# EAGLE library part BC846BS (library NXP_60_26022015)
Dual 65 V, 100 mA NPN/NPN general-purpose transistor AAL Eindhoven MK
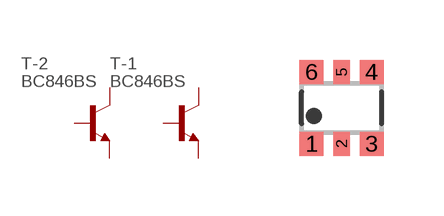
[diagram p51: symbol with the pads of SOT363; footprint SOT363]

Designator prefix T; gates -1=NPN -2=NPN

## BC846BS  [SOT363]
1  -1:E  pas
2  -1:B  pas
3  -2:C  pas
4  -2:E  pas
5  -2:B  pas
6  -1:C  pas

## Footprint SOT363 (pad centres in mm)
SOT363 Plastic surface-mounted package; 6 leads JEDEC: -- IEC: -- JEITA: SC-88
smd 0.6 x 0.6: 1 -0.75,-0.9; 3 0.75,-0.9; 4 0.75,0.9; 6 -0.75,0.9
smd 0.4 x 0.6: 2 0,-0.9; 5 0,0.9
